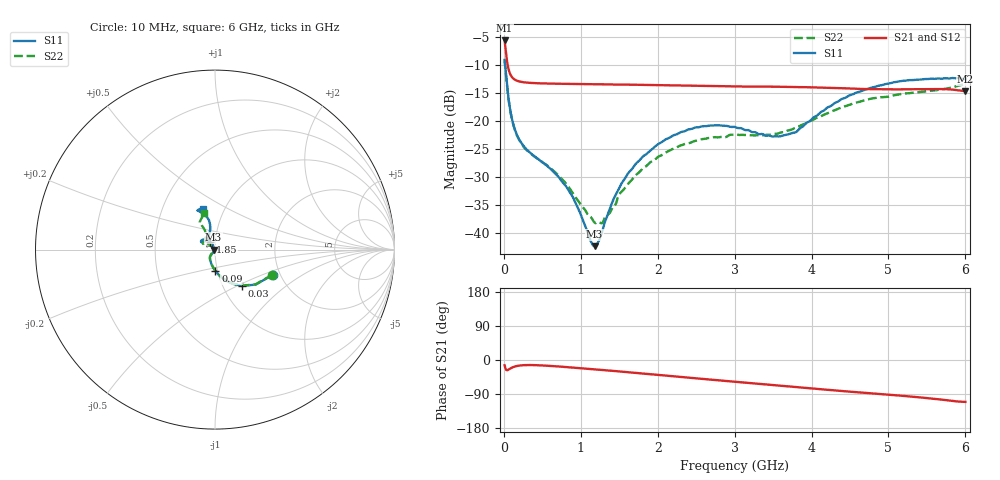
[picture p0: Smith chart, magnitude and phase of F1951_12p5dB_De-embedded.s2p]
! Integrated Device Technology
! Corporate Headquarters
! 6024 Silver Creek Valley Road
! San Jose, CA 95138  USA
! Phone:  1-408-284-8200
! Toll Free:  1-800-223-1366
! Webpage:  http://www.idt.com/
! Timing and RF Division
! 515 Groton Road, Suite 102
! Westford, MA 01886-6024
! Device:  F1951
! Description: 6-bit 0.5 dB Digital Step Attenuator
! Frequency:  100.0 -  4000.00 MHz
! Package:  4x4 mm Thin QFN Plastic Package: 24 pin
! Ports:  2 RF, 6 DC
!  Pin  1  = NC
!  Pin  2  = RF1  =  Port 1
!  Pin  3  = GND
!  Pin  4  = NC
!  Pin  5  = Serial Data Out (SDO)
!  Pin  6  = NC
!  Pin  7  = Reset Bar ( RSTb)
!  Pin  8  = Clock (CLK)
!  Pin  9  = Chip Select Bar (CSb)
!  Pin 10  = NC
!  Pin 11  = Serial Data In (SDI)
!  Pin 12  = NC
!  Pin 13  = NC
!  Pin 14  = VDD
!  Pin 15  = NC
!  Pin 16  = GND
!  Pin 17  = RF2  =  Port 2
!  Pin 18  = NC
!  Pin 19  = GND
!  Pin 20  = GND
!  Pin 21  = GND
!  Pin 22  = GND
!  Pin 23  = GND
!  Pin 24  = GND
! State:  25
! Atten State:  12.5 dB
! Voltage:  +3.30 Volts
! Current:  0.490 mA
! Data:  The device was measured on a F195X evaluation board which has
!  individual transmission lines to the RF pins.  Data was collected
!  de-embedded using a Automatic Fixture Removal [AFR] (Keysight Technologies).
!  The reference plane is the edge of the package pin.
! Misc:  Lot Code  1225BCA
!  Action Tracker AT0399
! Date Measured:  2018-09-13
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# GHz S dB R 50
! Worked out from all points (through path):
!   600 points, 10 MHz to 6 GHz, reference 50 ohm
!   highest |S21| = -5.65 dB at 10 MHz (marker M1); lowest = -14.7 dB at 6 GHz (marker M2)
!   group delay of S21, straight-line fit = 47.2 ps
!   lowest |S11| = -42.3 dB at 1.18 GHz (marker M3), VSWR 1.02, Z = 49.2 + j0.0419 ohm
!   |S11| at or under -10 dB: 16.45 MHz to end of sweep
!   |S22| runs from -38.2 to -9.2 dB; largest |S21 - S12| = 0.00042
!   S11 on the Smith chart (normalised r, x): 10 MHz: 1.82, -0.59; 30 MHz: 1.22, -0.53; 90 MHz: 0.98, -0.23; 1.85 GHz: 0.95, +0.08; 6 GHz: 0.80, +0.38
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0.01  -9.10 -23.8  -5.65 -14.0  -5.65 -14.0  -9.17 -23.9
0.03  -12.01 -53.6  -8.14 -25.9  -8.14 -26.0  -12.08 -53.8
0.06  -15.90 -76.4  -10.70 -25.6  -10.71 -25.6  -16.00 -76.7
0.09  -18.59 -89.0  -11.84 -21.7  -11.85 -21.7  -18.67 -89.5
0.16  -22.13 -106.3  -12.75 -16.3  -12.75 -16.3  -22.23 -106.4
0.26  -24.49 -117.9  -13.10 -13.7  -13.10 -13.6  -24.65 -118.7
0.72  -30.09 -124.4  -13.36 -17.2  -13.36 -17.3  -29.86 -129.2
0.88  -33.16 -125.6  -13.40 -19.7  -13.40 -19.7  -32.49 -131.2
1.01  -37.02 -132.0  -13.43 -21.8  -13.43 -21.8  -35.09 -136.3
1.18  -42.28 176.8  -13.45 -24.6  -13.46 -24.6  -38.08 -161.7
1.29  -39.09 133.4  -13.46 -26.5  -13.46 -26.5  -37.95 170.4
1.52  -31.37 116.4  -13.51 -30.5  -13.51 -30.5  -32.74 140.6
1.85  -25.91 121.3  -13.57 -36.6  -13.57 -36.5  -28.04 136.0
2.01  -24.08 126.3  -13.61 -39.5  -13.61 -39.5  -26.34 138.6
2.49  -21.15 140.5  -13.72 -48.2  -13.72 -48.2  -23.54 147.7
3.01  -21.08 151.3  -13.83 -57.4  -13.84 -57.3  -22.40 151.7
3.59  -22.73 130.3  -13.89 -67.7  -13.90 -67.7  -22.07 133.8
3.79  -22.02 115.2  -13.96 -71.3  -13.96 -71.3  -21.19 126.5
4.01  -19.57 105.4  -13.99 -75.2  -14.00 -75.2  -19.86 120.5
4.49  -15.45 101.8  -14.20 -83.5  -14.20 -83.4  -17.11 118.0
5.01  -13.31 109.9  -14.36 -91.6  -14.36 -91.6  -15.65 119.9
6  -12.53 106.0  -14.68 -110.5  -14.68 -110.5  -13.38 106.6
